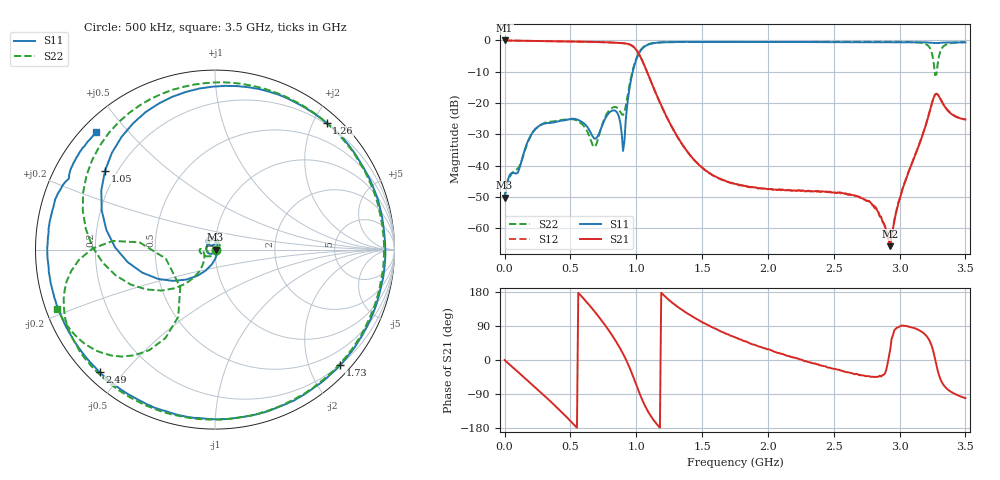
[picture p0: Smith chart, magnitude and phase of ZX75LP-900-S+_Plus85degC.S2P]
! Mini-Circuits
! S2P DATA File Format
! Type:LOW PASS FILTER
! Model: ZX75LP-900-S+
! All S Parameters are in dB deg format
! TEST CONDITIONS: INPUT POWER = 0 dBm @ Temperature = 85 deg C
! 401 Frequency points
# MHz S DB R 50
!FREQ	S11	S11_P	S21	S21_P	S12	S12_P	S22	S22_P
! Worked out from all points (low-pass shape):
!   401 points, 500 kHz to 3.5 GHz, reference 50 ohm
!   highest |S21| = -0.02 dB at 500 kHz (marker M1); lowest = -65.8 dB at 2.93 GHz (marker M2)
!   |S21| within 3 dB of the highest: start of sweep to 1 GHz
!   lowest |S11| = -50.3 dB at 500 kHz (marker M3), VSWR 1.01, Z = 50.3 + j0.0141 ohm
!   |S11| at or under -10 dB: start of sweep to 974 MHz
!   |S22| runs from -50.1 to -0.4 dB; largest |S21 - S12| = 0.0032
!   S11 on the Smith chart (normalised r, x): 500 kHz: 1.01, +0.00; 1.05 GHz: 0.15, +0.32; 1.26 GHz: 0.18, +2.20; 1.73 GHz: 0.20, -2.54; 2.49 GHz: 0.04, -0.43; 3.5 GHz: 0.04, +0.41
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0.5  -50.26 2.6  -0.02 -0.1  -0.02 -0.2  -50.14 2.5
300  -26.64 -169.1  -0.23 -93.4  -0.23 -93.4  -26.44 -176.3
590  -26.13 92.7  -0.41 166.0  -0.42 166.0  -26.81 67.3
680  -31.30 106.4  -0.50 129.7  -0.49 129.7  -34.06 -33.0
770  -24.55 139.5  -0.61 88.8  -0.61 88.8  -23.96 -145.7
910  -32.46 -58.3  -0.94 9.7  -0.92 9.6  -23.00 -146.2
990  -7.44 -162.4  -2.49 -55.9  -2.47 -55.9  -7.12 -149.7
1050  -2.45 144.3  -6.85 -108.5  -6.83 -108.7  -2.29 163.6
1170  -0.69 78.3  -18.90 -174.9  -18.96 -175.0  -0.69 100.8
1260  -0.53 48.6  -26.81 154.9  -26.87 155.1  -0.56 72.5
1460  -0.46 2.9  -39.03 108.2  -39.10 108.5  -0.53 29.2
1730  -0.46 -42.7  -45.53 62.8  -45.68 64.3  -0.52 -11.8
1760  -0.46 -47.0  -45.89 58.2  -45.91 59.3  -0.52 -15.7
2340  -0.54 -117.9  -48.29 -8.1  -48.19 -6.1  -0.48 -78.0
2490  -0.56 -133.3  -48.67 -22.6  -48.51 -21.7  -0.47 -91.6
2780  -0.59 -161.3  -51.84 -44.5  -51.75 -42.6  -0.46 -116.7
2920  -0.61 -174.4  -64.13 11.3  -64.36 6.8  -0.46 -128.8
2930  -0.61 -175.3  -65.77 29.5  -64.42 29.4  -0.47 -129.7
3200  -0.63 160.5  -27.00 65.3  -26.87 66.1  -1.23 -164.8
3270  -0.85 154.4  -17.31 2.4  -17.31 3.5  -11.10 -169.7
3330  -0.71 150.4  -20.28 -63.7  -20.20 -62.3  -2.03 -131.1
3500  -0.63 135.2  -25.29 -100.8  -25.18 -99.5  -0.55 -159.4
